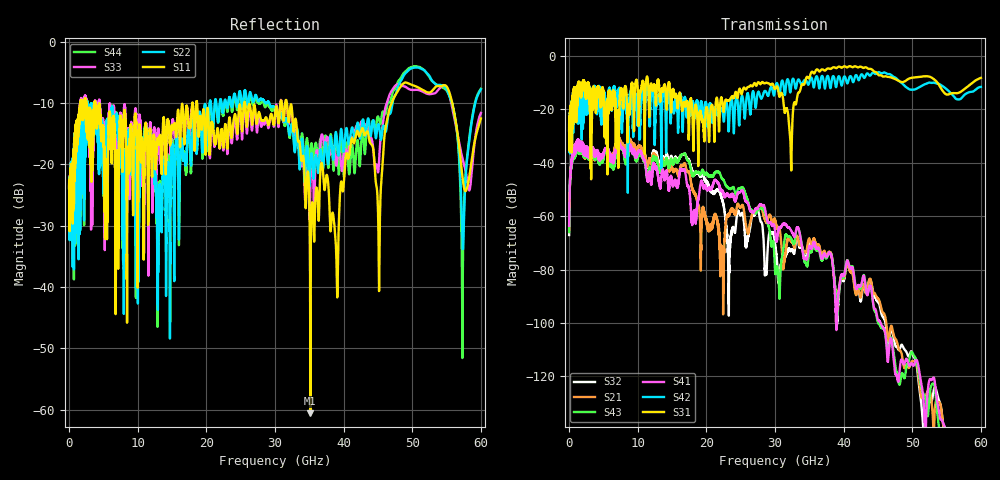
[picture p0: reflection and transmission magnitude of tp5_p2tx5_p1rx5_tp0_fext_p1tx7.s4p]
! 100G CR Analysis
! File: tp5_p2tx5_p1rx5_tp0_fext_p2tx7
! Description: 2m Cu Cable, OSFP, TP0-TP5
! Port Mapping
! Port1 -- P1RX5N
! Port2 -- P2TX7N
! Port3 -- P1RX5P
! Port4 -- P2TX7P
# GHz S MA R 50.00
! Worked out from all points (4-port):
!   6000 points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, 10 MHz to 60 GHz, reference 50 ohm
!   strongest paths, dB at 10 MHz, 15.01 GHz, 30.01 GHz, 45.01 GHz, 60 GHz:
!     S31: -27.9, -14.7, -12.4, -6.9, -8.2
!     S42: -27.9, -18.4, -12.9, -6.2, -11.6
!     S41: -63.6, -47.1, -65.2, -98.8, -175.4
!     S43: -66.0, -39.6, -80.3, -99.9, -177.9
!     S21: -65.2, -41.7, -61.6, -91.0, -193.4
!     S32: -67.1, -38.4, -70.8, -92.2, -179.9
!   lowest |S11| = -60.6 dB at 35.15 GHz (marker M1), VSWR 1.00, Z = 49.9 - j0.0169 ohm
!   |S11| at or under -10 dB: 4.391 GHz to 17.98 GHz (13.59 GHz wide, 121 % of centre); 18.65 GHz to 25.5 GHz (6.849 GHz wide, 31 % of centre); 31.74 GHz to 46.99 GHz (15.25 GHz wide, 38.7 % of centre)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
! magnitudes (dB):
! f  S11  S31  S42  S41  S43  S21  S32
! 10 MHz  -23.8  -27.9  -27.9  -63.6  -66.0  -65.2  -67.1
! 7.37 GHz  -13.4  -17.9  -13.1  -32.7  -32.7  -30.9  -31.1
! 22.28 GHz  -14.5  -16.3  -19.8  -50.6  -46.0  -74.2  -53.7
! 35.15 GHz  -60.6  -7.1  -8.5  -71.5  -73.2  -69.6  -70.6
! 51.29 GHz  -7.7  -7.8  -11.4  -122.3  -123.8  -127.5  -129.7
! 57.33 GHz  -22.2  -13.0  -15.3  -189.5  -174.5  -175.5  -175.7
! 60 GHz  -12.5  -8.2  -11.6  -175.4  -177.9  -193.4  -179.9
